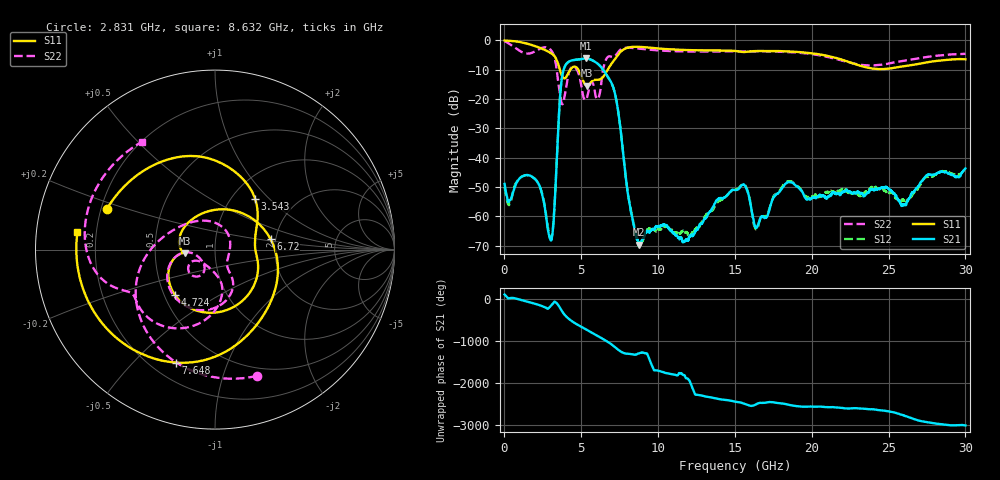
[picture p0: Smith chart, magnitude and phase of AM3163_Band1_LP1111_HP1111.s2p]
!Agilent Technologies,E8364B,MY43040894,A.07.50.67
!Agilent E8364B: A.07.50.67
!Date: Thursday, August 20, 2020 11:19:36
!Correction: S11(Full 2 Port(1,2))
!S21(Full 2 Port(1,2))
!S12(Full 2 Port(1,2))
!S22(Full 2 Port(1,2))
!S2P File: Measurements: S11, S21, S12, S22:
# Hz S  dB  R 50
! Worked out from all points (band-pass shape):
!   3201 points, 10 MHz to 30 GHz, reference 50 ohm
!   highest |S21| = -6.23 dB at 5.286 GHz (marker M1); lowest = -69.6 dB at 8.763 GHz (marker M2)
!   |S21| within 3 dB of the highest: 3.904 GHz to 6.305 GHz (2.401 GHz wide, 47 % of centre)
!   lowest |S11| = -15.5 dB at 5.371 GHz (marker M3), VSWR 1.40, Z = 35.7 - j1.47 ohm
!   |S11| at or under -10 dB: 3.605 GHz to 4.294 GHz (689.4 MHz wide, 17.5 % of centre); 4.804 GHz to 6.723 GHz (1.919 GHz wide, 33.3 % of centre)
!   |S22| runs from -21.8 to -0.3 dB; largest |S21 - S12| = 0.0046
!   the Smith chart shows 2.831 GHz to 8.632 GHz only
!   S11 on the Smith chart (normalised r, x): 2.831 GHz: 0.22, +0.17; 3.543 GHz: 1.28, +0.83; 4.724 GHz: 0.57, -0.32; 6.72 GHz: 1.88, +0.24; 7.648 GHz: 0.30, -0.67; 8.632 GHz: 0.13, +0.06
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1e7  -0.08 -4.6  -48.96 96.0  -49.98 9.1  -0.34 -11.5
1.097138e9  -0.71 -72.4  -46.60 -34.8  -46.58 -35.3  -3.93 -164.9
1.893747e9  -1.82 -125.6  -46.86 -114.5  -46.90 -113.2  -4.05 73.8
2.830934e9  -3.84 159.3  -64.66 117.0  -63.88 -55.5  -2.60 -71.7
3.149578e9  -4.84 120.9  -64.69 -121.4  -64.32 137.4  -4.39 -127.6
3.543197e9  -8.87 51.6  -25.71 -177.8  -25.67 -178.5  -15.88 100.4
4.724053e9  -9.45 -131.6  -6.62 104.8  -6.62 105.0  -10.12 -148.4
5.014581e9  -12.37 -166.4  -6.39 45.3  -6.38 45.3  -15.93 -174.8
5.286366e9  -15.31 -173.6  -6.23 -9.6  -6.22 -9.7  -20.33 -138.3
5.370712e9  -15.50 -173.2  -6.25 -26.8  -6.25 -26.9  -19.55 -125.4
6.045488e9  -13.50 130.5  -7.90 -164.5  -7.90 -164.6  -20.07 -124.5
6.720262e9  -10.03 10.6  -12.38 50.0  -12.47 50.2  -5.74 -124.8
7.648078e9  -3.53 -109.1  -34.65 161.8  -34.69 162.8  -2.90 -179.6
8.632125e9  -2.24 172.9  -68.03 117.4  -68.02 -152.3  -2.78 124.2
8.763331e9  -2.26 164.9  -69.63 132.5  -70.07 -7.2  -2.86 118.1
1.000979e10  -2.80 101.0  -63.63 83.7  -64.38 76.0  -3.46 66.1
1.228716e10  -3.40 9.9  -66.52 -16.1  -65.76 -47.0  -3.85 -14.7
1.5005e10  -3.64 -73.5  -50.99 65.4  -50.82 68.6  -3.80 -91.7
1.638267e10  -3.68 -104.4  -64.02 0.9  -64.42 0.7  -3.80 -125.4
2.000958e10  -4.45 163.1  -53.76 -51.6  -53.25 -51.3  -4.72 136.6
2.500479e10  -9.69 -62.6  -50.57 -167.7  -51.89 -168.3  -7.97 -92.6
3e10  -6.50 104.2  -43.68 -141.7  -43.97 -130.0  -4.64 102.3
